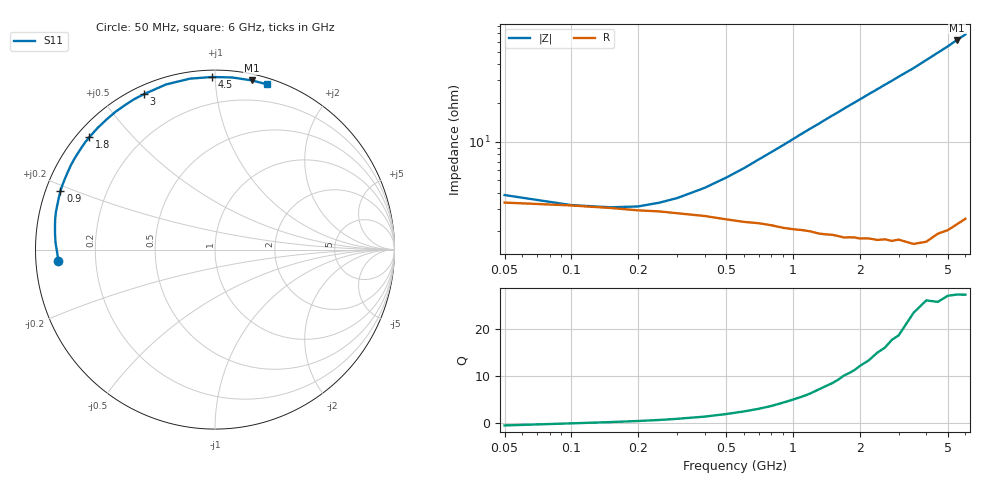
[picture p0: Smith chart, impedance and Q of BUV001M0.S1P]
! Infineon Technologies  Discrete & RF Semiconductors
! BB 833
! Si Tuning Diode in SOD323
! VR =
! S-Parameters:  June  1999
# GHz  S  MA  R  50
!  f  S11
! GHz  MAG  ANG
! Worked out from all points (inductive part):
!   34 points, 50 MHz to 6 GHz, reference 50 ohm
!   read as one part to ground: L = 1.64 nH near 800 MHz
!   highest Q = 27.2 at 5.5 GHz (marker M1), where L = 1.79 nH
!   S11 on the Smith chart (normalised r, x): 50 MHz: 0.07, -0.04; 900 MHz: 0.04, +0.18; 1.8 GHz: 0.04, +0.38; 3 GHz: 0.03, +0.64; 4.5 GHz: 0.04, +0.98; 6 GHz: 0.05, +1.37
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0.05  0.8745 -175.7
0.1  0.8802 -179.2
0.15  0.8852 178.9
0.2  0.8898 177.4
0.3  0.8952 174.6
0.5  0.9062 169.4
0.6  0.9105 166.9
0.8  0.9166 161.8
0.9  0.9206 159.3
1  0.9232 156.8
1.1  0.925 154.3
1.3  0.9306 149.6
1.4  0.9325 147.2
1.6  0.936 142.7
1.7  0.9385 140.4
1.8  0.9391 138.2
2  0.942 134.0
2.2  0.9438 129.8
2.4  0.947 125.9
2.6  0.9483 122.0
2.8  0.9514 118.4
3  0.9522 114.7
3.5  0.9598 106.5
4  0.9626 98.3
4.5  0.9618 90.9
5  0.9638 84.3
5.5  0.9647 77.8
6  0.9656 72.4
